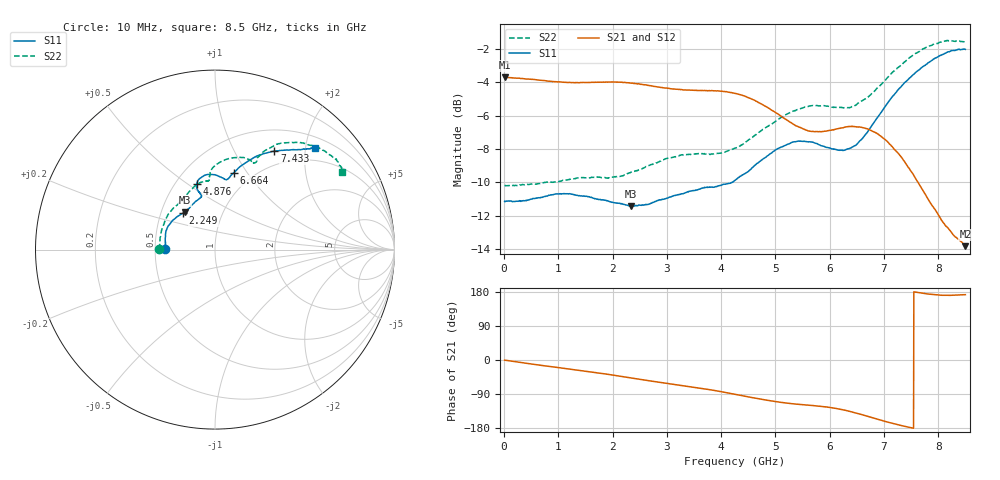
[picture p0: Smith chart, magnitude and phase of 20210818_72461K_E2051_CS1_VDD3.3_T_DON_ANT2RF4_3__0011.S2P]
!Agilent Technologies,E5071C,MY46417908,A.11.23
!Date: Wed Aug 18 14:34:21 2021
!Data & Calibration Information:
!Freq	S11:SOLT2(ON)	S21:SOLT2(ON)	S12:SOLT2(ON)	S22:SOLT2(ON)
!PortZ  Port1:50+j0  Port2:50+j0
!Above PortZ is port z conversion or system Z0 setting when saving the data.
!When reading, reference impedance value at option line is always used.
# Hz S dB R 50
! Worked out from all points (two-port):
!   1601 points, 10 MHz to 8.5 GHz, reference 50 ohm
!   highest |S21| = -3.69 dB at 10 MHz (marker M1); lowest = -13.8 dB at 8.5 GHz (marker M2)
!   |S21| within 3 dB of the highest: start of sweep to 5.436 GHz; 6.288 GHz to 6.531 GHz (242.5 MHz wide, 3.78 % of centre)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
!   lowest |S11| = -11.4 dB at 2.334 GHz (marker M3), VSWR 1.73, Z = 32.9 + j14.7 ohm
!   |S11| at or under -10 dB: start of sweep to 4.207 GHz
!   |S22| runs from -10.2 to -1.5 dB; largest |S21 - S12| = 0.0016
!   S11 on the Smith chart (normalised r, x): 10 MHz: 0.57, +0.00; 2.249 GHz: 0.65, +0.29; 4.876 GHz: 0.63, +0.55; 6.664 GHz: 0.82, +0.87; 7.433 GHz: 0.79, +1.47; 8.5 GHz: 0.72, +2.19
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1e7  -11.15 179.6  -3.69 -0.4  -3.69 -0.3  -10.17 179.8
9.22675e8  -10.72 160.3  -3.95 -18.6  -3.95 -18.6  -9.99 156.5
1.426769e9  -10.82 148.2  -4.01 -28.0  -4.01 -27.9  -9.72 141.8
2.249238e9  -11.36 131.0  -4.01 -45.3  -4.01 -45.3  -9.52 121.9
2.334138e9  -11.44 129.1  -4.05 -47.2  -4.05 -47.2  -9.41 120.4
2.843538e9  -11.09 118.2  -4.28 -58.4  -4.28 -58.4  -8.79 110.1
3.591719e9  -10.42 104.9  -4.49 -73.8  -4.49 -73.9  -8.27 97.9
4.255e9  -9.89 104.7  -4.66 -90.4  -4.66 -90.4  -7.96 94.6
4.875831e9  -8.37 105.4  -5.56 -106.9  -5.55 -106.8  -6.62 90.0
5.321556e9  -7.59 98.3  -6.50 -115.5  -6.51 -115.5  -5.74 80.6
5.671769e9  -7.59 90.4  -6.95 -120.0  -6.96 -120.0  -5.40 72.8
5.889325e9  -7.84 85.5  -6.94 -123.2  -6.96 -123.2  -5.40 69.0
6.260762e9  -8.08 80.7  -6.71 -131.9  -6.71 -132.0  -5.52 66.1
6.457094e9  -7.81 79.0  -6.66 -138.9  -6.66 -139.0  -5.41 64.9
6.664038e9  -7.12 76.3  -6.77 -147.1  -6.76 -147.1  -4.98 65.3
6.865675e9  -6.17 72.5  -7.06 -155.6  -7.06 -155.6  -4.38 63.8
7.088538e9  -5.14 67.4  -7.65 -164.7  -7.66 -164.8  -3.64 60.8
7.433444e9  -3.87 58.9  -9.04 -176.7  -9.04 -176.7  -2.64 53.9
7.810188e9  -2.84 50.5  -10.99 174.1  -10.97 174.0  -1.83 44.8
8.048969e9  -2.38 47.5  -12.22 170.9  -12.20 170.9  -1.59 38.7
8.356731e9  -2.04 45.7  -13.39 171.3  -13.36 171.3  -1.52 33.2
8.5e9  -2.02 45.5  -13.84 172.4  -13.81 172.3  -1.62 31.5
